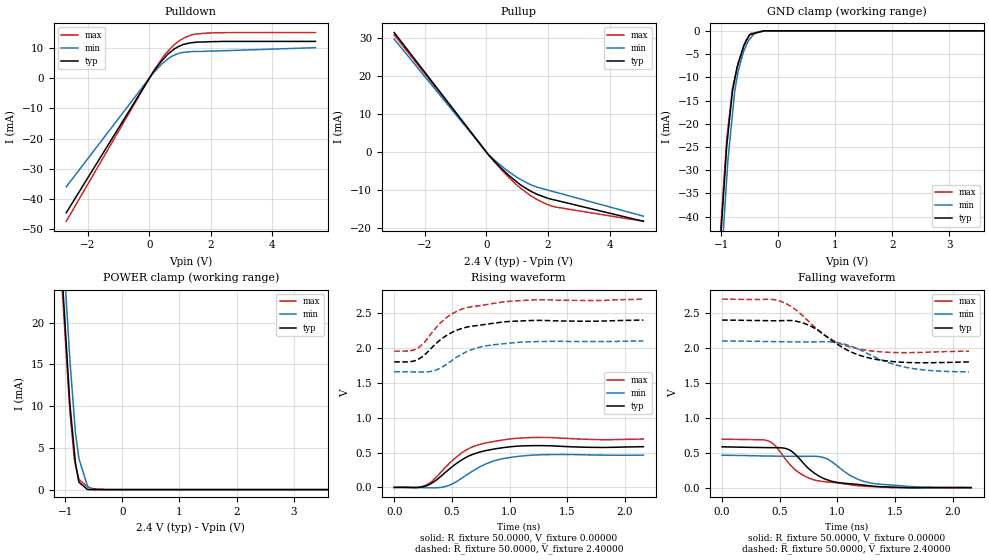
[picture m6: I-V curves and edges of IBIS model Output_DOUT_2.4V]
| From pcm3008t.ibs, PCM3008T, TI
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[Model] Output_DOUT_2.4V
Model_type Output
Vref  = 0.00000V
Cref  = 2.00000pF
Vmeas = 1.20000V
C_comp  1.57000pF 1.57000pF 1.57000pF
[Model spec]
|   typ   min   max
Vmeas  1.2000V  1.0500V  1.3500V
| variable   typ   min   max
[Voltage Range]   2.40000V  2.10000V  2.70000V
[POWER Clamp Reference]  2.40000V  2.10000V  2.70000V
[Pullup Reference]   2.40000V  2.10000V  2.70000V
[Pulldown Reference]   0.00000V  0.00000V  0.00000V
[GND Clamp Reference]   0.00000V  0.00000V  0.00000V
[Temperature Range]   25   85   -25
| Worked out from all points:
|   slope of the pulldown table from 0 to 0.36 V, typ, clamps not added: 69.1 ohm
|   slope of the pullup table from 0 to 0.36 V, typ, clamps not added: 112 ohm
|   GND clamp passes 1 mA (typ) near -0.51 V on its own axis
|   POWER clamp passes 1 mA (typ) near -0.76 V on its own axis
|   rising waveform, R_fixture 50.0000, V_fixture 0.00000: 20-80 % time 296ps typ, 298ps min, 286ps max; typ from 0 V to 0.584 V
|   falling waveform, R_fixture 50.0000, V_fixture 0.00000: 20-80 % time 263ps typ, 275ps min, 265ps max; typ from 0.584 V to 0 V
|   falling waveform, R_fixture 50.0000, V_fixture 2.40000: 20-80 % time 347ps typ, 388ps min, 335ps max; typ from 2.4 V to 1.8 V
|   rising waveform, R_fixture 50.0000, V_fixture 2.40000: 20-80 % time 312ps typ, 307ps min, 303ps max; typ from 1.8 V to 2.4 V
[GND Clamp]
-2.7V     -360.7mA   -372.9mA   -353.1mA
-2.1V     -248.6mA   -259.1mA   -243.1mA
-901.3mV  -24.85mA   -31.82mA   -23.31mA
-881.1mV  -22.46mA   -27.99mA   -21.12mA
-800.4mV  -12.94mA   -17.92mA   -12.39mA
-760mV    -10.41mA   -12.88mA   -10.17mA
-699.4mV  -7.061mA   -8.601mA   -6.83mA
-603.1mV  -3.209mA   -4.363mA   -3.438mA
-481.7mV  -785.3uA   -1.537mA   -577.3uA
-360.4mV  -372.5uA   -239.7uA   -286.6uA
-180.2mV  0A         0A         0A
5.4V      0A         0A         0A
[Pulldown]
-2.7V     -44.54mA   -35.97mA   -47.39mA
101.9mV   1.645mA    1.305mA    1.762mA
400.8mV   5.703mA    4.649mA    6.333mA
603.1mV   7.945mA    6.36mA     8.873mA
840.9mV   9.86mA     7.739mA    11.36mA
1.119V    11.21mA    8.514mA    13.24mA
1.301V    11.59mA    8.741mA    14.07mA
1.74V     11.95mA    8.845mA    14.82mA
2.539V    12.14mA    9.099mA    15.07mA
5.4V      12.14mA    10.07mA    15.07mA
[Pullup]
-3V       31.42mA    29.69mA    30.82mA
77.7mV    -897.6uA   -771.3uA   -863.3uA
497.8mV   -4.454mA   -3.758mA   -4.765mA
761.3mV   -6.422mA   -5.409mA   -6.978mA
1.079V    -8.507mA   -7.122mA   -9.351mA
1.337V    -9.846mA   -8.249mA   -10.94mA
1.701V    -11.34mA   -9.397mA   -12.81mA
2.201V    -12.63mA   -10.5mA    -14.45mA
5.1V      -18.26mA   -16.9mA    -18.21mA
[POWER Clamp]
-3V       245mA      251.2mA    238.6mA
-1.079V   28.39mA    33.74mA    26.93mA
-1.019V   21.56mA    26.87mA    20.25mA
-937.9mV  12.45mA    17.72mA    11.35mA
-917.8mV  10.18mA    15.45mA    9.253mA
-841.9mV  4.669mA    8.633mA    3.748mA
-821.6mV  3.196mA    6.811mA    2.942mA
-761.3mV  902.7uA    3.744mA    1.242mA
-609mV    0A         401.5uA    298.3uA
-518mV    0A         0A         120.7uA
-226.5mV  0A         0A         0A
5.1V      0A         0A         0A
[Rising Waveform]
R_fixture = 50.0000
V_fixture = 0.00000
V_fixture_min = 0.00000
V_fixture_max = 0.00000
0s        0V         0V         0V
200ps     -1.603mV   -1.164mV   601uV
280ps     23.87mV    -3.914mV   37.5mV
440ps     211.2mV    11.96mV    282.1mV
580ps     389mV      126.9mV    490.9mV
680ps     473.9mV    234.4mV    582.8mV
800ps     530mV      341mV      639.9mV
940ps     569.4mV    411.6mV    680.3mV
1.2ns     598.9mV    463.1mV    715.1mV
2.16ns    584mV      462.9mV    694.1mV
[Falling Waveform]
R_fixture = 50.0000
V_fixture = 0.00000
V_fixture_min = 0.00000
V_fixture_max = 0.00000
0s        584mV      462.9mV    694.1mV
400ps     573mV      452.7mV    668.4mV
460ps     572.6mV    451.3mV    601.5mV
580ps     542.5mV    449mV      345mV
700ps     358.5mV    448mV      180.1mV
820ps     186.2mV    447.8mV    101.8mV
980ps     80.52mV    334mV      70.75mV
1.14ns    50.99mV    148mV      34.55mV
1.28ns    26.44mV    69.07mV    16.44mV
2.16ns    0V         0V         0V
[Falling Waveform]
R_fixture = 50.0000
V_fixture = 2.40000
V_fixture_min = 2.10000
V_fixture_max = 2.70000
0s        2.4V       2.1V       2.7V
420ps     2.391V     2.092V     2.698V
520ps     2.392V     2.09V      2.661V
620ps     2.39V      2.088V     2.571V
760ps     2.321V     2.087V     2.365V
980ps     2.075V     2.082V     2.094V
1.18ns    1.902V     1.986V     1.988V
1.4ns     1.82V      1.816V     1.943V
1.58ns    1.794V     1.728V     1.933V
2.14ns    1.8V       1.659V     1.954V
[Rising Waveform]
R_fixture = 50.0000
V_fixture = 2.40000
V_fixture_min = 2.10000
V_fixture_max = 2.70000
0s        1.8V       1.659V     1.954V
120ps     1.8V       1.658V     1.956V
200ps     1.829V     1.655V     1.993V
260ps     1.897V     1.655V     2.077V
340ps     2.028V     1.671V     2.244V
460ps     2.185V     1.772V     2.444V
640ps     2.302V     1.954V     2.581V
800ps     2.34V      2.032V     2.622V
1.1ns     2.388V     2.083V     2.68V
2.16ns    2.4V       2.1V       2.7V
[Ramp]
| variable typ min max
dV/dt_r 349.889m/326.348p 276.743m/326.268p 416.426m/307.716p
dV/dt_f 360.333m/347.202p 265.712m/388.409p 449.307m/335.384p
R_load = 50.0000Ohms
